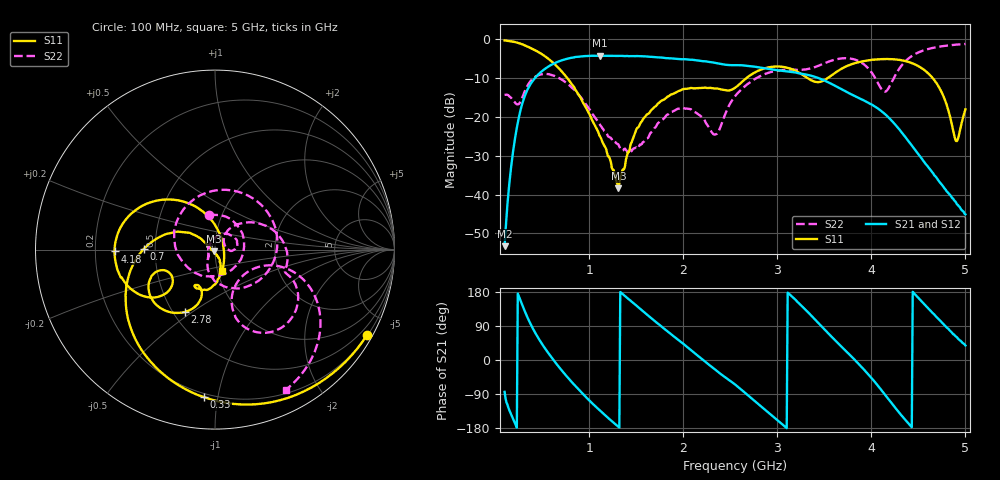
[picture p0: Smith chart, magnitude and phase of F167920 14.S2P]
!  2-Port S-parameters saved by WinCal
! VAR MeasName=S-Parameters (CALIBRATED_DATA) read from VNA (N5242A)
! VAR MeasDate=2016-11-22 9:54:16
! VAR NAME=F167920 14
! VAR FILENAME=F167920 14.S2P
! VAR DATE=2016-11-22 9:54:16
! VAR PHYS_PORTS=1,2
# Hz S DB R 50
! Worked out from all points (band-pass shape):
!   491 points, 100 MHz to 5 GHz, reference 50 ohm
!   highest |S21| = -4.18 dB at 1.11 GHz (marker M1); lowest = -53.3 dB at 100 MHz (marker M2)
!   |S21| within 3 dB of the highest: 553.5 MHz to 2.803 GHz (2.25 GHz wide, 134 % of centre)
!   lowest |S11| = -38.4 dB at 1.31 GHz (marker M3), VSWR 1.02, Z = 49.2 - j0.857 ohm
!   |S11| at or under -10 dB: 768.2 MHz to 2.669 GHz (1.901 GHz wide, 111 % of centre); 3.326 GHz to 3.533 GHz (207.1 MHz wide, 6.04 % of centre); 4.654 GHz to end of sweep
!   |S22| runs from -29.2 to -1.2 dB; largest |S21 - S12| = 0.0017
!   S11 on the Smith chart (normalised r, x): 100 MHz: 0.22, -3.82; 330 MHz: 0.18, -0.91; 700 MHz: 0.43, +0.00; 2.78 GHz: 0.57, -0.47; 4.18 GHz: 0.28, -0.01; 5 GHz: 1.05, -0.25
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1e8  -0.25 -29.3  -53.29 -84.1  -52.93 -83.5  -14.28 99.5
2e8  -0.61 -58.0  -27.24 -160.5  -27.20 -160.7  -15.97 -6.7
3.3e8  -1.68 -94.3  -13.64 119.9  -13.63 120.0  -12.58 165.1
4.5e8  -3.10 -124.7  -9.21 61.3  -9.19 61.4  -9.31 74.7
7e8  -8.03 179.5  -5.43 -25.2  -5.43 -25.3  -10.23 -29.5
9.2e8  -15.55 146.1  -4.33 -86.3  -4.33 -86.3  -15.16 -91.0
1.11e9  -24.84 145.9  -4.18 -132.4  -4.17 -132.4  -21.82 -122.5
1.31e9  -38.39 -133.6  -4.24 -176.2  -4.24 -176.2  -27.06 -148.7
1.5e9  -23.25 -66.3  -4.27 144.0  -4.27 144.0  -27.83 139.9
1.74e9  -16.37 -80.6  -4.62 94.2  -4.61 94.2  -21.37 73.3
2.14e9  -12.57 -111.9  -5.36 14.2  -5.35 14.2  -18.95 1.9
2.35e9  -12.64 -118.8  -6.10 -27.8  -6.09 -27.8  -24.40 28.4
2.55e9  -12.47 -108.6  -6.61 -64.5  -6.60 -64.6  -14.64 48.8
2.78e9  -8.25 -115.9  -7.09 -112.6  -7.07 -112.7  -9.92 23.7
3.08e9  -7.15 -146.3  -8.16 -175.5  -8.14 -175.7  -7.81 -6.9
3.37e9  -10.63 -156.0  -9.41 114.8  -9.39 114.7  -7.35 -19.1
3.85e9  -5.94 -152.2  -14.90 -6.3  -14.88 -6.5  -5.40 -59.8
4.18e9  -5.04 -179.0  -20.03 -102.9  -20.03 -103.1  -12.65 -28.5
4.19e9  -5.05 -179.9  -20.27 -105.9  -20.28 -106.3  -12.25 -25.2
4.65e9  -9.89 123.3  -34.33 124.2  -34.34 124.5  -2.18 -43.0
4.9e9  -26.16 16.9  -42.00 61.8  -42.14 61.7  -1.33 -58.3
5e9  -18.01 -71.3  -45.09 38.4  -45.14 38.7  -1.15 -63.3
